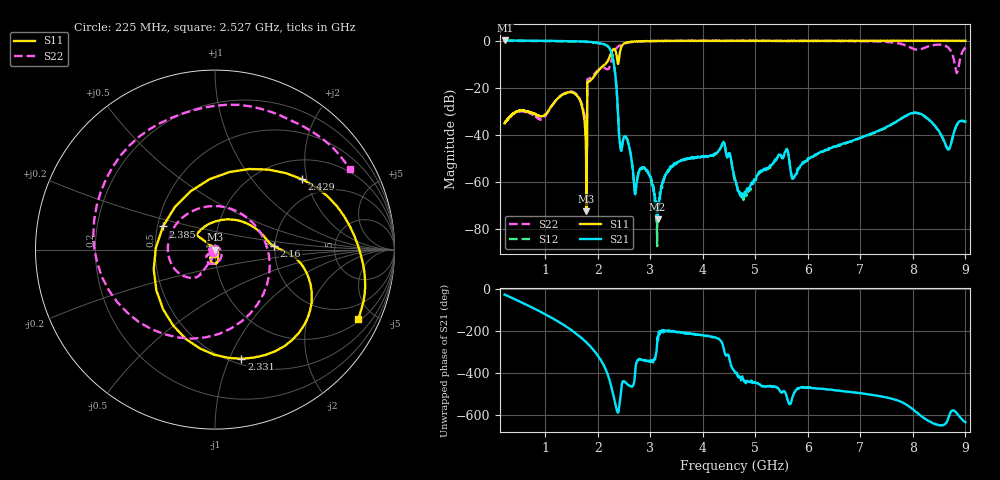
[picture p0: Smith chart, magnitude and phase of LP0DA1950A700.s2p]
!Agilent Technologies,E8358A,US41080443,A.07.50.56
!Agilent E8358A: A.07.50.56
!Date: Wednesday, May 04, 2016 15:06:30
!Correction: S11(Full 2 Port(1,2))
!S21(Full 2 Port(1,2))
!S12(Full 2 Port(1,2))
!S22(Full 2 Port(1,2))
!S2P File: Measurements: S11, S21, S12, S22:Log Frequency Sweep
# Hz S  dB  R 50
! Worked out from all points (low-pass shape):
!   1601 points, 225 MHz to 9 GHz, reference 50 ohm
!   highest |S21| = 0.03 dB at 227.1 MHz (marker M1); lowest = -76.1 dB at 3.138 GHz (marker M2)
!   |S21| within 3 dB of the highest: start of sweep to 2.214 GHz
!   lowest |S11| = -72.6 dB at 1.784 GHz (marker M3), VSWR 1.00, Z = 50 - j0.00825 ohm
!   |S11| at or under -10 dB: start of sweep to 2.145 GHz
!   |S22| runs from -35.1 to -0.1 dB; largest |S21 - S12| = 0.019
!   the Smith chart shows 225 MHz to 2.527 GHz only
!   S11 on the Smith chart (normalised r, x): 225 MHz: 0.99, -0.03; 2.16 GHz: 1.98, +0.09; 2.331 GHz: 0.55, -1.11; 2.385 GHz: 0.54, +0.15; 2.429 GHz: 1.46, +1.87; 2.527 GHz: 1.11, -4.05
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2.25e8  -35.24 -104.9  0.02 -26.0  -0.13 -25.9  -35.09 -126.9
2.270846e8  -35.19 -105.2  0.03 -26.3  -0.14 -26.1  -35.00 -127.6
9.310556e8  -32.23 -100.6  -0.10 -111.2  -0.26 -111.0  -33.40 54.6
1.687749e9  -27.08 -123.7  -0.35 127.0  -0.51 127.2  -26.51 -144.8
1.783769e9  -72.65 -20.7  -0.42 105.1  -0.58 105.3  -33.45 -94.3
1.833809e9  -17.30 124.6  -0.58 92.4  -0.74 92.5  -16.17 -120.1
2.159959e9  -9.64 3.3  -1.94 -29.3  -2.11 -29.4  -12.11 118.3
2.330709e9  -4.07 -76.4  -14.13 175.2  -14.23 175.4  -3.96 -159.1
2.385069e9  -9.97 156.0  -31.24 130.0  -31.38 130.0  -2.59 135.4
2.429468e9  -4.11 39.0  -45.00 -158.0  -45.20 -157.8  -2.00 94.1
2.52658e9  -1.04 -26.0  -40.79 -85.7  -40.93 -86.1  -1.17 30.8
3.138009e9  -0.15 -100.1  -76.13 131.7  -71.85 107.5  -0.16 -86.7
3.152512e9  -0.17 -101.4  -68.87 126.2  -73.03 134.9  -0.17 -88.2
3.401725e9  -0.11 -112.7  -53.43 157.4  -53.78 159.5  -0.10 -104.8
4.343458e9  -0.22 -138.8  -45.47 112.0  -45.60 113.1  -0.15 -145.1
4.622431e9  -0.15 -143.8  -59.51 -41.3  -60.71 -39.4  -0.07 -155.3
6.081681e9  -0.10 -173.7  -49.41 -113.6  -49.60 -113.2  -0.19 144.4
7.553438e9  -0.16 166.2  -36.26 -160.5  -36.21 -160.5  -0.65 66.5
8.094374e9  -0.05 161.7  -30.77 126.6  -30.99 126.8  -3.94 -84.1
8.321445e9  -0.16 159.8  -34.04 86.9  -34.17 86.7  -2.34 -178.7
8.574632e9  -0.11 157.9  -41.80 70.0  -41.81 69.9  -1.98 122.4
9e9  -0.10 155.7  -34.47 84.2  -34.66 84.4  -2.80 179.3
